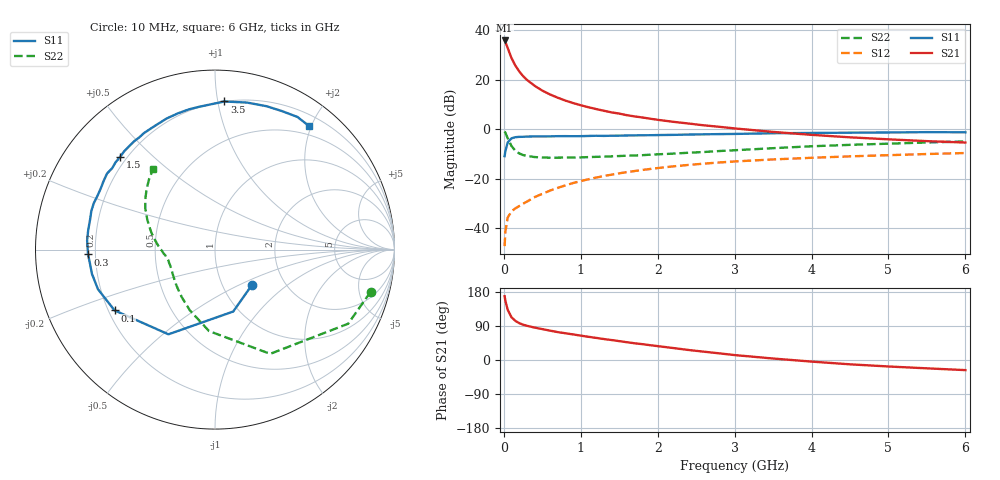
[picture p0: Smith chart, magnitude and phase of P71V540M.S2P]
! SIEMENS Small Signal Semiconductors
! BFP196
! Si NPN RF Bipolar Junction Transistor in SOT143
! VCE = 1.5 V  IC = 40 mA
! Common Emitter S-Parameters:  May  1996
# GHz  S  MA  R  50
!  f  S11  S21  S12  S22
! GHz  MAG  ANG  MAG  ANG  MAG  ANG  MAG  ANG
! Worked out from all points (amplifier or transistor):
!   36 points, 10 MHz to 6 GHz, reference 50 ohm
!   highest |S21| = 35.9 dB at 10 MHz (marker M1)
!   |S21| within 3 dB of that: start of sweep to 49.6 MHz
!   unconditionally stable (mu >= 1): 466.5 MHz to 4.645 GHz
!   at 250 MHz: K = 0.82, MSG = 25.8 dB, |S12| = -30.2 dB
!   at 1.4 GHz: K = 1.10, MAG = 10.7 dB, |S12| = -18.4 dB
!   at 6 GHz: K = 1.00, MSG = 2.1 dB, |S12| = -9.7 dB
!   S11 on the Smith chart (normalised r, x): 10 MHz: 1.37, -0.59; 100 MHz: 0.22, -0.27; 300 MHz: 0.17, -0.02; 1.5 GHz: 0.17, +0.40; 3.5 GHz: 0.20, +1.04; 6 GHz: 0.36, +1.97
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0.01  0.2849 -43.6  62.29 168.3  0.0043 78.8  0.8983 -15.2
0.02  0.3596 -73.6  58.2 156.4  0.0085 69.6  0.8492 -29.1
0.05  0.5385 -118.8  43.93 132.5  0.0163 53.4  0.6572 -62.1
0.1  0.6541 -148.8  27.39 112.7  0.0218 45.7  0.4551 -94.2
0.15  0.6884 -161.3  19.27 103.2  0.025 45.8  0.3659 -112.6
0.2  0.6989 -168.9  14.77 97.3  0.0278 48.2  0.3233 -124.9
0.25  0.7013 -174.0  11.84 93.2  0.031 50.5  0.2994 -134.1
0.3  0.7078 -177.8  9.949 90.3  0.0342 53.7  0.2873 -140.3
0.4  0.7143 175.9  7.539 85.5  0.0422 56.7  0.2729 -149.3
0.5  0.7147 171.4  6.031 81.5  0.0492 58.8  0.267 -155.2
0.6  0.7155 166.8  5.035 77.5  0.0572 60.1  0.2648 -159.3
0.7  0.7219 162.6  4.334 73.6  0.0649 60.5  0.2653 -162.4
0.8  0.7231 159.1  3.788 70.6  0.0729 60.3  0.2662 -164.7
1.1  0.7289 148.4  2.775 61.2  0.0969 58.6  0.2724 -170.2
1.5  0.7388 135.8  2.065 49.8  0.128 54.1  0.2862 -175.4
1.7  0.7493 129.3  1.811 44.1  0.1424 51.6  0.2938 -178.4
2.2  0.7667 115.7  1.41 31.6  0.1767 44.4  0.3199 175.3
3  0.8009 96.1  1.035 13.0  0.2224 32.7  0.3746 163.4
3.5  0.8268 86.4  0.88 3.9  0.2443 25.8  0.4126 156.1
4.5  0.849 70.2  0.684 -11.4  0.2819 13.9  0.4818 143.6
5.5  0.8702 58.1  0.573 -22.0  0.3144 3.1  0.5383 133.0
6  0.865 52.6  0.536 -26.7  0.3292 -2.7  0.5646 127.7
